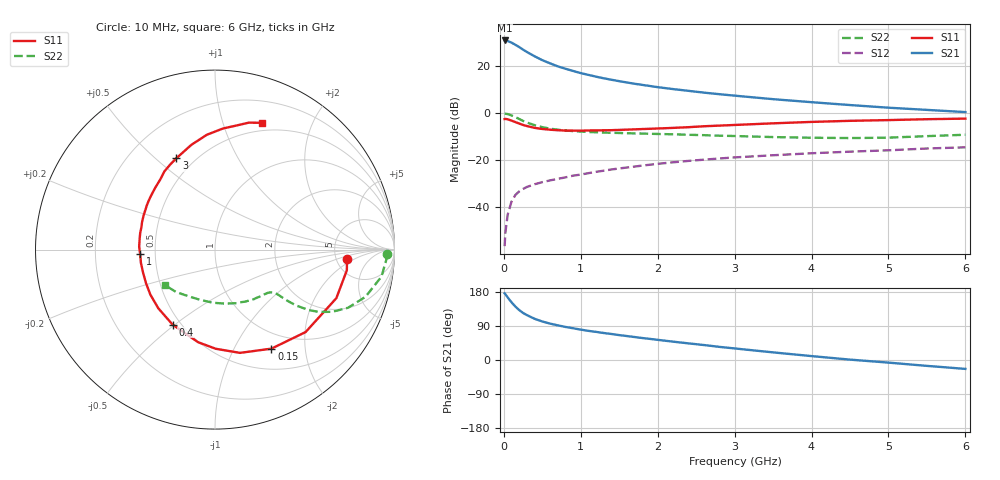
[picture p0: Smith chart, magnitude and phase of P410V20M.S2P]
! SIEMENS Small Signal Semiconductors
! BFP182
! Si NPN RF Bipolar Junction Transistor in SOT143
! VCE = 10 V  IC = 20 mA
! Common Emitter S-Parameters:  March  1996
# GHz  S  MA  R  50
!  f  S11  S21  S12  S22
! GHz  MAG  ANG  MAG  ANG  MAG  ANG  MAG  ANG
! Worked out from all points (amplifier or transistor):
!   36 points, 10 MHz to 6 GHz, reference 50 ohm
!   highest |S21| = 30.6 dB at 10 MHz (marker M1)
!   |S21| within 3 dB of that: start of sweep to 208.8 MHz
!   unconditionally stable (mu >= 1): 951.8 MHz to 5.754 GHz
!   at 250 MHz: K = 0.44, MSG = 29.5 dB, |S12| = -32.3 dB
!   at 1.4 GHz: K = 1.10, MAG = 17.0 dB, |S12| = -24.0 dB
!   at 6 GHz: K = 0.98, MSG = 7.5 dB, |S12| = -14.6 dB
!   S11 on the Smith chart (normalised r, x): 10 MHz: 6.28, -1.42; 150 MHz: 0.77, -1.43; 400 MHz: 0.45, -0.49; 1 GHz: 0.41, -0.02; 3 GHz: 0.40, +0.59; 6 GHz: 0.41, +1.35
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0.01  0.7372 -4.0  34.01 175.9  0.0015 74.0  0.9578 -1.6
0.02  0.7436 -8.9  33.88 173.7  0.0029 80.3  0.9558 -3.5
0.05  0.7283 -21.8  33.06 165.2  0.007 81.1  0.9398 -9.2
0.1  0.6826 -42.3  30.54 152.2  0.0132 68.2  0.8789 -17.4
0.15  0.6352 -60.3  27.54 141.0  0.0182 62.7  0.8092 -23.6
0.2  0.592 -76.4  24.61 131.6  0.0217 58.5  0.7385 -28.0
0.25  0.5525 -89.6  21.71 124.1  0.0244 55.1  0.674 -31.0
0.3  0.5244 -100.4  19.39 118.5  0.0269 52.0  0.6224 -32.8
0.4  0.4801 -119.5  15.72 108.7  0.0307 50.3  0.5472 -34.6
0.5  0.4546 -134.0  13 101.6  0.034 49.5  0.4964 -35.2
0.6  0.439 -145.1  11.17 96.1  0.037 49.8  0.4623 -35.4
0.7  0.4274 -154.2  9.627 91.5  0.04 50.3  0.4393 -35.5
0.8  0.4207 -162.5  8.579 87.3  0.0429 50.7  0.4223 -35.7
1  0.4179 -176.7  6.92 80.2  0.0492 51.4  0.4004 -36.6
1.1  0.4229 177.7  6.345 76.9  0.0527 50.9  0.3928 -37.3
1.5  0.434 159.6  4.673 65.7  0.0663 50.3  0.3738 -41.3
2.2  0.4791 134.1  3.177 48.4  0.0895 46.1  0.3506 -52.0
3  0.5524 113.0  2.307 30.5  0.1136 39.4  0.3223 -67.8
3.5  0.5984 102.7  1.943 20.1  0.1262 34.7  0.3062 -79.5
4.5  0.6759 86.3  1.459 1.0  0.1504 26.2  0.2917 -106.0
5.5  0.7319 75.1  1.152 -15.5  0.1755 18.7  0.3205 -132.4
6  0.7527 69.8  1.035 -23.5  0.1857 13.9  0.343 -145.0
